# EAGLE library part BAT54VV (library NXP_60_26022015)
Schottky barrier triple diode Planar Schottky barrier triple diode with an integrated guard ring for stress protection. Three electrically isolated Schottky barrier diodes, encapsulated in a SOT666 ultra small SMD plastic package. AAL Eindhoven MK
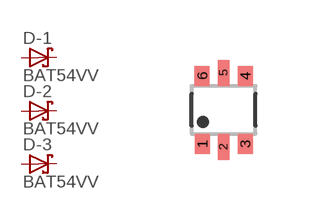
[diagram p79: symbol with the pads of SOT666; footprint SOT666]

Designator prefix D; gates -1=DIODE_SCHOTTKY -2=DIODE_SCHOTTKY -3=DIODE_SCHOTTKY

## BAT54VV  [SOT666]
1  -1:A  pas
2  -2:A  pas
3  -3:A  pas
4  -3:K  pas
5  -2:K  pas
6  -1:K  pas

## Footprint SOT666 (pad centres in mm)
SOT 666 Reflow soldering foorprint Source: Philips - BAS70_1PS7XSB70_SER_8.pdf
smd 0.375 x 0.5: 1 -0.537,-0.85; 3 0.538,-0.85; 4 0.538,0.85; 6 -0.538,0.85
smd 0.3 x 0.65: 2 0,-0.925; 5 0,0.925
